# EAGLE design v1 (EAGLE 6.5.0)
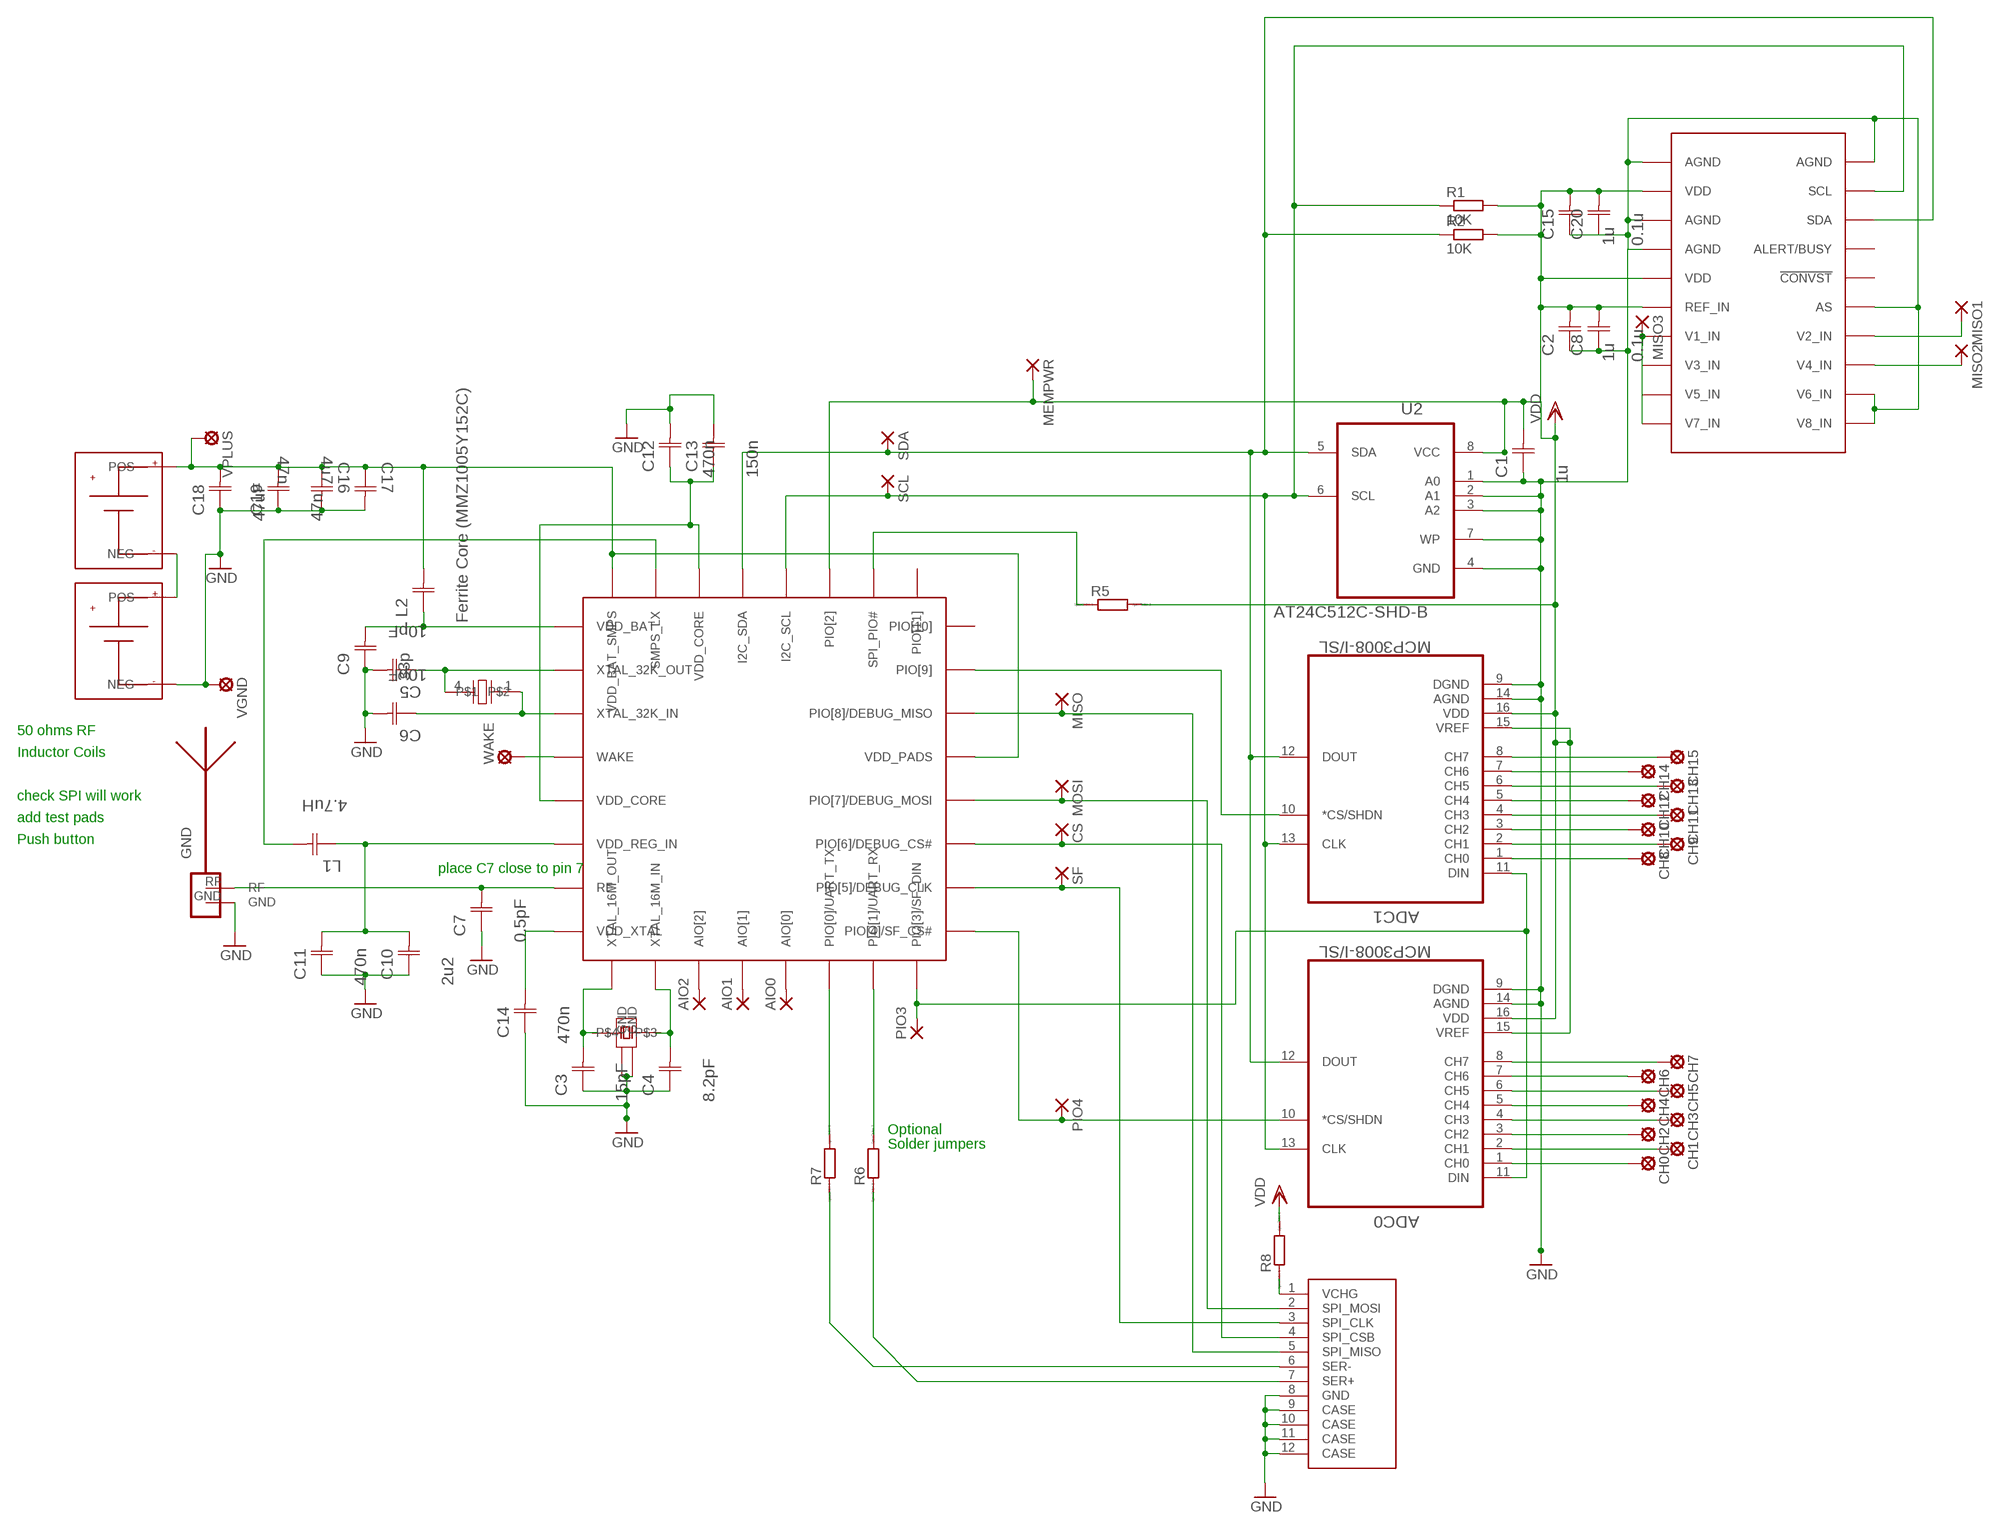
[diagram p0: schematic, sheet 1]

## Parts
ADC0  MCP3008-I/SL  [SOIC127P600X175-16N]
ADC1  MCP3008-I/SL  [SOIC127P600X175-16N]
AIO0  1,6/0,8  [1,6/0,8]
AIO1  1,6/0,8  [1,6/0,8]
AIO2  1,6/0,8  [1,6/0,8]
C1  1u  UQCL2A100JAT2A/500  [CAPC1005X60N]
C2  1u  UQCL2A100JAT2A/500  [CAPC1005X60N]
C3  15pF  UQCL2A150JAT2A/500  [CAPC1005X60N]
C4  8.2pF  UQCL2A8R2CAT2A/500  [CAPC1005X60N]
C5  10pF  UQCL2A100JAT2A/500  [CAPC1005X60N]
C6  10pF  UQCL2A100JAT2A/500  [CAPC1005X60N]
C7  0.5pF  UQCL2A0R5BAT2A/500  [CAPC1005X60N]
C8  0.1u  UQCL2A100JAT2A/500  [CAPC1005X60N]
C9  33p  UQCL2A100JAT2A/500  [CAPC1005X60N]
C10  2u2  UQCL2A100JAT2A/500  [CAPC1005X60N]
C11  470n  UQCL2A100JAT2A/500  [CAPC1005X60N]
C12  470n  UQCL2A100JAT2A/500  [CAPC1005X60N]
C13  150n  UQCL2A100JAT2A/500  [CAPC1005X60N]
C14  470n  UQCL2A100JAT2A/500  [CAPC1005X60N]
C15  1u  UQCL2A100JAT2A/500  [CAPC1005X60N]
C16  47n  UQCL2A1R0BAT2A/500  [CAPC1005X60N]
C17  4u7  UQCL2A1R0BAT2A/500  [CAPC1005X60N]
C18  47uF  0805AA100MAT1A  [CAPC2012X130N]
C19  47n  0805AA100MAT1A  [CAPC2012X130N]
C20  0.1u  UQCL2A100JAT2A/500  [CAPC1005X60N]
CH0  LSP10  [LSP10]
CH1  LSP10  [LSP10]
CH2  LSP10  [LSP10]
CH3  LSP10  [LSP10]
CH4  LSP10  [LSP10]
CH5  LSP10  [LSP10]
CH6  LSP10  [LSP10]
CH7  LSP10  [LSP10]
CH8  LSP10  [LSP10]
CH9  LSP10  [LSP10]
CH10  LSP10  [LSP10]
CH11  LSP10  [LSP10]
CH12  LSP10  [LSP10]
CH13  LSP10  [LSP10]
CH14  LSP10  [LSP10]
CH15  LSP10  [LSP10]
CS  1,6/0,8  [1,6/0,8]
GND  ANTENNA_1LEFT  [SWRA117D_LEFT]
L1  4.7uH  12107C102JAT2A  [CAPC3225X127N]
L2  Ferrite Core (MMZ1005Y152C)  UQCL2A100JAT2A/500  [CAPC1005X60N]
MEMPWR  1,6/0,8  [1,6/0,8]
MISO  1,6/0,8  [1,6/0,8]
MISO1  1,6/0,8  [1,6/0,8]
MISO2  1,6/0,8  [1,6/0,8]
MISO3  1,6/0,8  [1,6/0,8]
MOSI  1,6/0,8  [1,6/0,8]
PIO3  1,6/0,8  [1,6/0,8]
PIO4  1,6/0,8  [1,6/0,8]
R1  10K  R-EU_R0402  [R0402]
R2  10K  R-EU_R0402  [R0402]
R5  RR1206  [R1206]
R6  RR1206  [R1206]
R7  RR1206  [R1206]
R8  RR1206  [R1206]
SCL  1,6/0,8  [1,6/0,8]
SDA  1,6/0,8  [1,6/0,8]
SF  1,6/0,8  [1,6/0,8]
U2  AT24C512C-SHD-B  [SOIC127P798X216-8N]
U$1  CSR1010A05-IQQM-R  [CSR1010A05-IQQM-R]
U$2  8PIN_SMT_CONNECTOR  [8PIN_SMT_CONNECTOR]
U$3  TSX3225  [TSX3225]
U$4  SSP-T7-F  [SSP-T7-F]
U$5  BATTERY_2996  [BATTERY_2996]
U$6  BATTERY_2996  [BATTERY_2996]
U$7  AD7997  [AD7997]
VGND  LSP10  [LSP10]
VPLUS  Vrail  LSP10  [LSP10]
WAKE  Vrail  LSP10  [LSP10]

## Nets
GND: ADC0.9(DGND) ADC0.14(AGND) ADC1.9(DGND) ADC1.14(AGND) C1.2(C1) C2.2(C1) C3.2(C1) C4.2(C1) C5.1(C2) C6.1(C2) C7.2(C1) C8.2(C1) C9.2(C1) C10.2(C1) C11.2(C1) C12.1(C2) C13.1(C2) C14.2(C1) C15.2(C1) C16.1(C2) C17.1(C2) C18.1(C1) C19.1(C1) U2.1(A0) U2.2(A1) U2.3(A2) U2.4(GND) U2.7(WP) U$2.8(GND) U$2.9(CASE) U$2.10(CASE) U$2.11(CASE) U$2.12(CASE) U$3.2(GND) U$3.4(GND) U$5.NEG U$7.P$01(AGND) U$7.P$03(AGND) U$7.P$04(AGND) U$7.P$015(AS) U$7.P$020(AGND) VGND.MP
N$1: ADC0.8(CH7) CH7.MP
N$2: ADC0.7(CH6) CH6.MP
N$3: ADC0.6(CH5) CH5.MP
N$4: ADC0.5(CH4) CH4.MP
N$5: ADC0.4(CH3) CH3.MP
N$6: ADC0.3(CH2) CH2.MP
N$7: ADC0.2(CH1) CH1.MP
N$8: ADC0.1(CH0) CH0.MP
N$9: ADC1.8(CH7) CH15.MP
N$10: ADC1.7(CH6) CH14.MP
N$11: ADC1.6(CH5) CH13.MP
N$12: ADC1.5(CH4) CH12.MP
N$13: ADC1.4(CH3) CH11.MP
N$14: ADC1.3(CH2) CH10.MP
N$15: ADC1.2(CH1) CH9.MP
N$16: ADC1.1(CH0) CH8.MP
N$17: AIO2.1(P) U$1.AIO[2]
N$18: MISO.1(P) U$1.PIO[8]/DEBUG_MISO U$2.5(SPI_MISO)
N$19: L1.2(C2) U$1.SMPS_LX
N$20: R7.1 U$2.6(SER-)
N$23: ADC0.11(DIN) ADC1.11(DIN) PIO3.1(P) U$1.PIO[3]/SF_DIN
N$24: ADC1.10(*CS/SHDN) U$1.PIO[9]
N$25: ADC0.10(*CS/SHDN) PIO4.1(P) U$1.PIO[4]/SF_CS#
N$26: C5.2(C1) U$1.XTAL_32K_OUT U$4.4
N$27: C6.2(C1) U$1.XTAL_32K_IN U$4.1
N$29: C3.1(C2) U$1.XTAL_16M_OUT
N$30: C4.1(C2) U$1.XTAL_16M_IN
N$31: CS.1(P) U$1.PIO[6]/DEBUG_CS# U$2.4(SPI_CSB)
N$32: C9.1(C2) L2.2(C1) U$1.VDD_BAT
N$33: AIO1.1(P) U$1.AIO[1]
N$34: C16.2(C1) C17.2(C1) C18.2(C2) C19.2(C2) L2.1(C2) U$1.VDD_BAT_SMPS U$1.VDD_PADS U$6.POS@1(POS) VPLUS.MP
N$35: C14.1(C2) U$1.VDD_XTAL
N$36: R6.1 U$2.7(SER+)
N$37: R7.2 U$1.PIO[0]/UART_TX
N$38: R6.2 U$1.PIO[1]/UART_RX
N$39: C10.1(C2) C11.1(C2) L1.1(C1) U$1.VDD_REG_IN
N$40: R8.1 U$2.1(VCHG)
N$41: AIO0.1(P) U$1.AIO[0]
N$43: C7.1(C2) U$1.RF
N$45: R5.1 U$1.SPI_PIO#
N$48: U$5.POS@1(POS) U$6.NEG
N$49: U$1.WAKE WAKE.MP
N$50: MOSI.1(P) U$1.PIO[7]/DEBUG_MOSI U$2.2(SPI_MOSI)
N$51: SF.1(P) U$1.PIO[5]/DEBUG_CLK U$2.3(SPI_CLK)
N$86: MISO1.1(P) U$7.P$014(V2_IN)
N$87: MISO2.1(P) U$7.P$013(V4_IN)
N$88: MISO3.1(P) U$7.P$07(V1_IN) U$7.P$010(V7_IN)
N$90: U$7.P$011(V8_IN) U$7.P$012(V6_IN)
SCL: ADC0.13(CLK) ADC1.13(CLK) R1.1 SCL.1(P) U2.6(SCL) U$1.I2C_SCL U$7.P$019(SCL)
SDA: ADC0.12(DOUT) ADC1.12(DOUT) R2.1 SDA.1(P) U2.5(SDA) U$1.I2C_SDA U$7.P$018(SDA)
VDD: ADC0.15(VREF) ADC0.16(VDD) ADC1.15(VREF) ADC1.16(VDD) C1.1(C2) C2.1(C2) C8.1(C2) C15.1(C2) C20.1(C2) MEMPWR.1(P) R1.2 R2.2 R5.2 R8.2 U2.8(VCC) U$1.PIO[2] U$7.P$02(VDD) U$7.P$05(VDD) U$7.P$06(REF_IN)
VDD_CORE: C12.2(C1) C13.2(C1) U$1.VDD_CORE U$1.VDD_CORE@1(VDD_CORE)
Unconnected: C20.2(C1) GND.GND GND.RF U$1.PIO[10] U$1.PIO[11] U$3.1 U$3.3 U$7.P$08(V3_IN) U$7.P$09(V5_IN) U$7.P$016(!CONVST) U$7.P$017(ALERT/BUSY)

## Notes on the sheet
- 50 ohms RF
- Inductor Coils
- check SPI will work
- add test pads
- Push button
- place C7 close to pin 7
- Optional
- Solder jumpers

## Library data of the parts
ADC0 ADC1 = Microchip_By_element14_Batch_1:MCP3008-I/SL: 10BIT ADC, 8 CH, SPI, SMD; MPN: MCP3008-I/SL; OC_FARNELL: 1292241; OC_NEWARK: 19C7201; PACKAGE: SOIC16; SUPPLIER: Microchip
AIO0 AIO1 AIO2 CS MEMPWR MISO MISO1-MISO3 MOSI PIO3 PIO4 SCL SDA SF = wirepad:1,6/0,8: THROUGH-HOLE PAD
C1 C2 C8-C15 C20 L2 = AVX_By_element14_Batch_1:UQCL2A100JAT2A/500: Capacitor 0402; MPN: UQCL2A100JAT2A/500; OC_FARNELL: -; OC_NEWARK: 32T8791; SUPPLIER: AVX; TOLERANCE: ±5%; VALUE: 10pF; VOLTAGERATING: 200V
C3 = AVX_By_element14_Batch_1:UQCL2A150JAT2A/500: Capacitor 0402; MPN: UQCL2A150JAT2A/500; OC_FARNELL: -; OC_NEWARK: 32T8795; SUPPLIER: AVX; TOLERANCE: ±5%; VOLTAGERATING: 200V
C4 = AVX_By_element14_Batch_1:UQCL2A8R2CAT2A/500: Capacitor 0402; MPN: UQCL2A8R2CAT2A/500; OC_FARNELL: -; OC_NEWARK: 32T8828; SUPPLIER: AVX; TOLERANCE: ±.25 pF; VOLTAGERATING: 200V
C5 C6 = AVX_By_element14_Batch_1:UQCL2A100JAT2A/500: Capacitor 0402; MPN: UQCL2A100JAT2A/500; OC_FARNELL: -; OC_NEWARK: 32T8791; SUPPLIER: AVX; TOLERANCE: ±5%; VOLTAGERATING: 200V
C7 = AVX_By_element14_Batch_1:UQCL2A0R5BAT2A/500: Capacitor 0402; MPN: UQCL2A0R5BAT2A/500; OC_FARNELL: -; OC_NEWARK: 32T8767; SUPPLIER: AVX; TOLERANCE: ±.1 pF; VOLTAGERATING: 200V
C16 C17 = AVX_By_element14_Batch_1:UQCL2A1R0BAT2A/500: Capacitor 0402; MPN: UQCL2A1R0BAT2A/500; OC_FARNELL: -; OC_NEWARK: 32T8778; SUPPLIER: AVX; TOLERANCE: ±.1 pF; VALUE: 1pF; VOLTAGERATING: 200V
C18 C19 = AVX_By_element14_Batch_1:0805AA100MAT1A: Capacitor 0805; MPN: 0805AA100MAT1A; OC_FARNELL: -; OC_NEWARK: 18M6883; SUPPLIER: AVX; TOLERANCE: ±20%; VALUE: 10pF; VOLTAGERATING: 1000V (1kV)
CH0 CH1-CH15 VGND VPLUS WAKE = solpad:LSP10: SOLDER PAD
GND = ant-planar-1:ANTENNA_1
L1 = AVX_By_element14_Batch_1:12107C102JAT2A: Capacitor 1210; MPN: 12107C102JAT2A; OC_FARNELL: -; OC_NEWARK: 56J0850; SUPPLIER: AVX; TOLERANCE: ±5%; VALUE: 1000PF; VOLTAGERATING: 500V
R1 R2 = rcl:R-EU_: RESISTOR, European symbol
R5-R8 = eagle-ltspice:R: RESISTOR, European symbol; SPICEMODEL: NONE; SPICEPREFIX: R
U2 = ATMEL-AT24C512C-SHD-B:AT24C512C-SHD-B: EEPROM, SERIAL, 512K (64KX8), 8SOIC-Wide; MPN: AT24C512C-SHD-B; OC_FARNELL: 1972003; OC_NEWARK: 68T4124; PACKAGE: 8SOIC-Wide; SUPPLIER: ATMEL
U$1 = CSR1010A05:CSR1010A05-IQQM-R
U$2 = MINI_SMT_8_PIN_CONNECTOR:8PIN_SMT_CONNECTOR
U$3 = TSX3225:TSX3225
U$4 = SSP-T7-F:SSP-T7-F
U$5 U$6 = BATTERY_2996:BATTERY_2996
U$7 = AD7997:AD7997

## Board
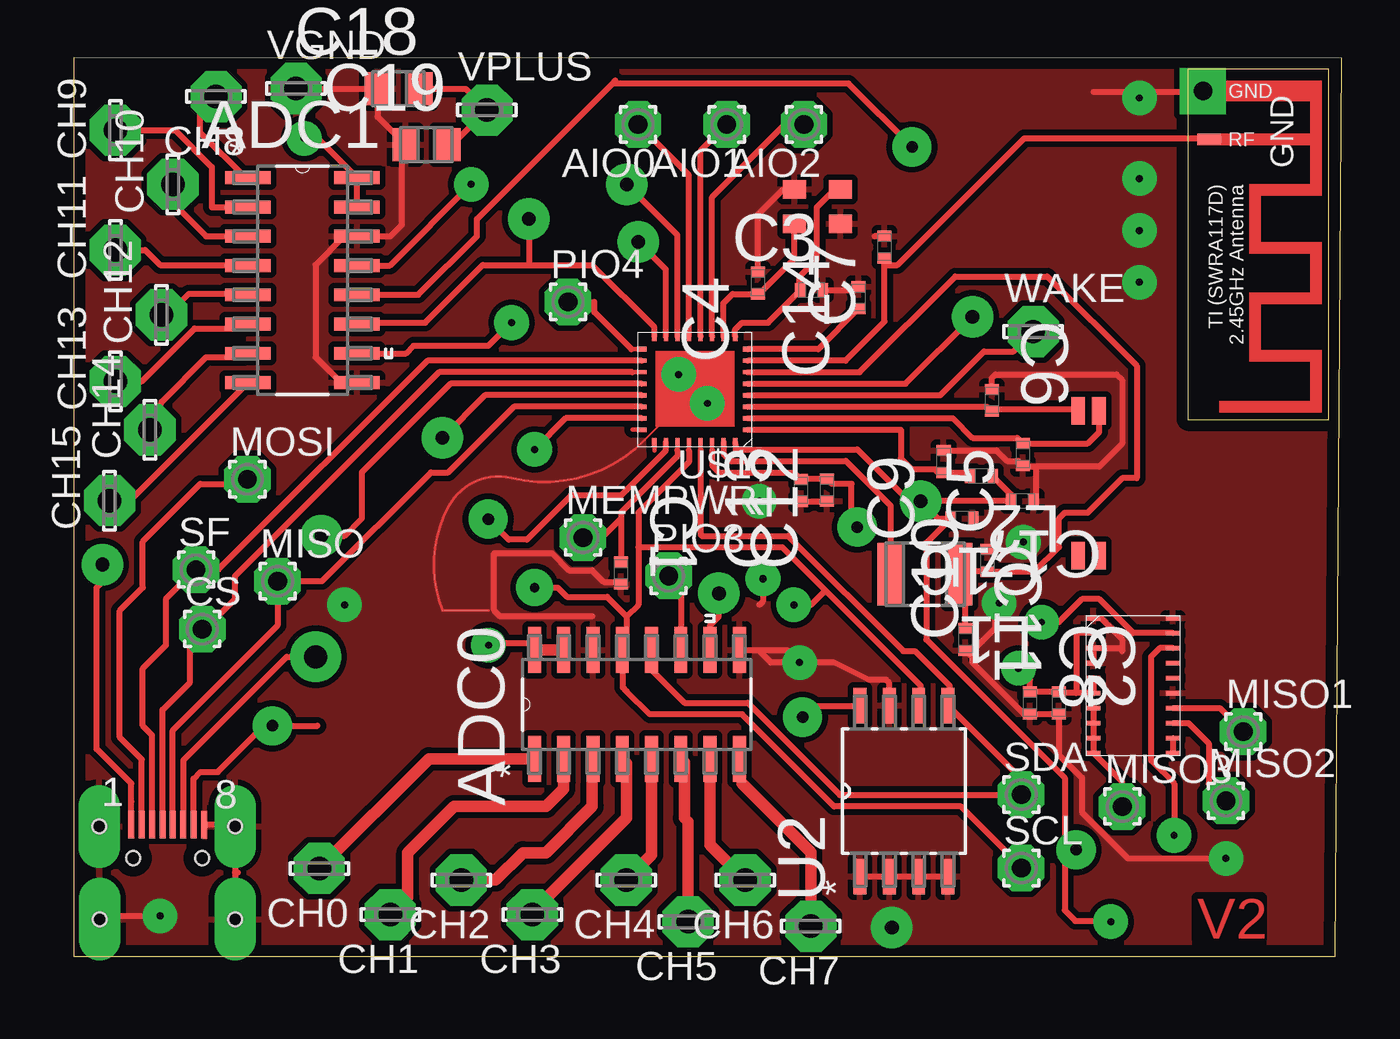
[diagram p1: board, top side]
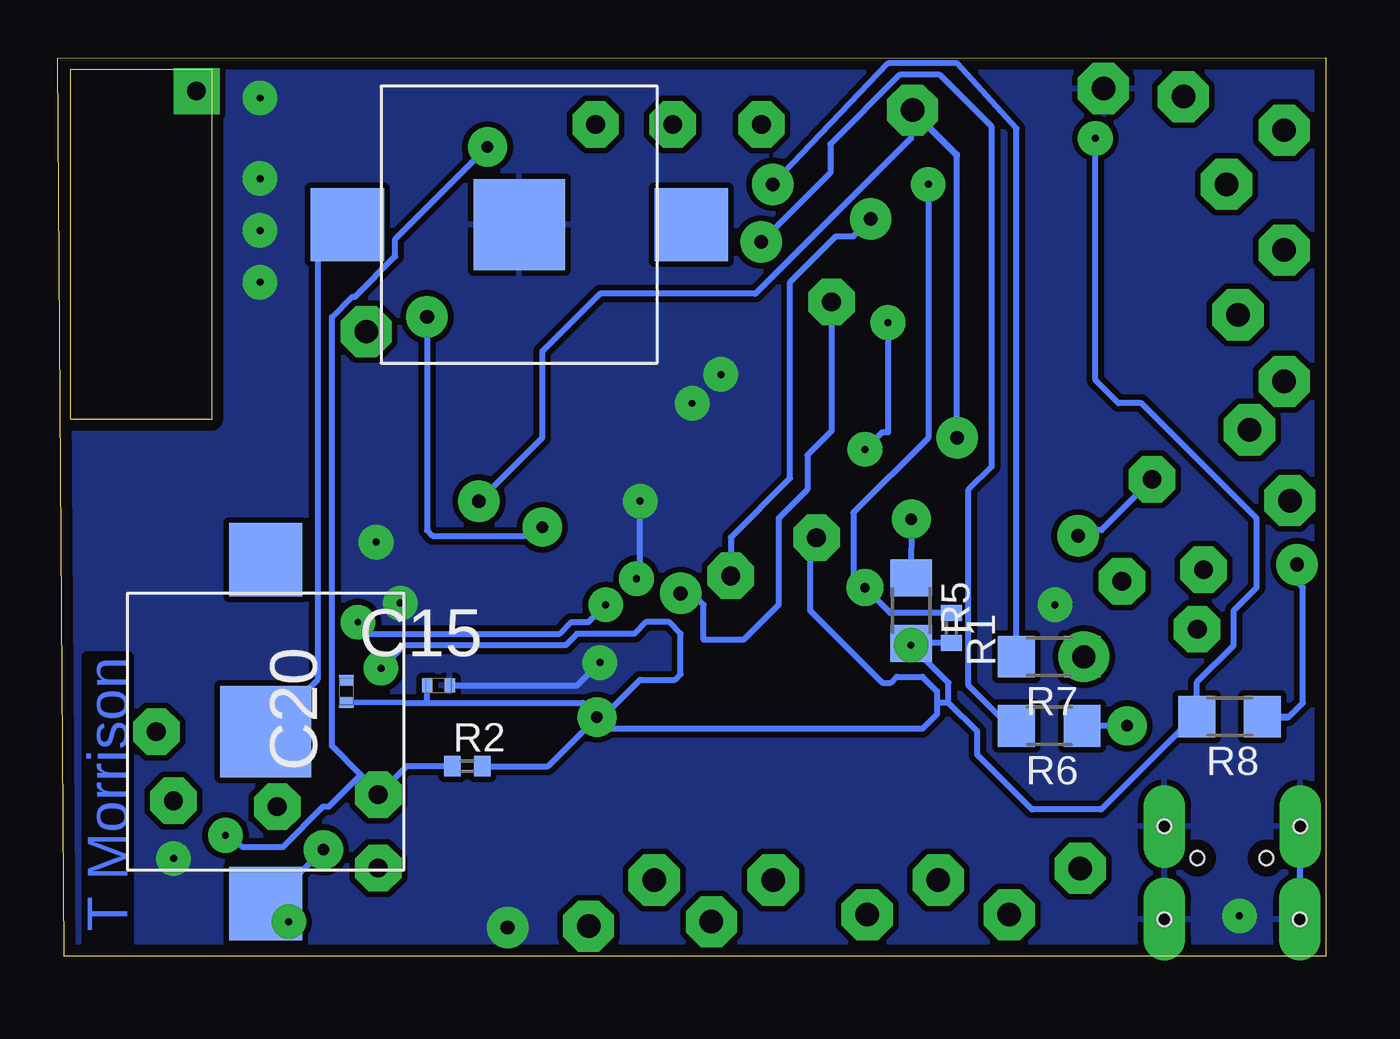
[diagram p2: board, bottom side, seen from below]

Size 55.04 x 38.99 mm. Coordinates in mm from the lower left corner, seen from the top.
Outline: 0.01,0 54.76,0 55.04,38.98 0,38.99 0.01,0
Copper layers (1*16): Top 0.035mm / dielectric 1.5mm / Bottom 0.035mm
Design rules "DRC *": minimum track width 0.25mm, minimum drill 0.5mm, track to track 0.25mm, track to pad 0.25mm, pad to pad 0.15mm, via to via 0.25mm, smd to smd 0.15mm, copper to edge 0.5mm, drill to drill 0.4mm, minimum pad ring 0.6mm, minimum via ring 0.6mm, stop-mask expansion 4mil, vias tented up to drill 0mil, thermal gap 10mil

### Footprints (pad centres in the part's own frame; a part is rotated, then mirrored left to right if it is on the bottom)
SOIC127P600X175-16N = smd 1.981 x 0.559: 1 -2.362,4.445; 2 -2.362,3.175; 3 -2.362,1.905; 4 -2.362,0.635; 5 -2.362,-0.635; 6 -2.362,-1.905; 7 -2.362,-3.175; 8 -2.362,-4.445; 9 2.362,-4.445; 10 2.362,-3.175; 11 2.362,-1.905; 12 2.362,-0.635; 13 2.362,0.635; 14 2.362,1.905; 15 2.362,3.175; 16 2.362,4.445
1,6/0,8 = drill 0.813 pad 1.6 octagon: 1 0,0
CAPC1005X60N = smd 0.457 x 0.61: 1 -0.483,0; 2 0.483,0
CAPC2012X130N = smd 1.118 x 1.448: 1 -0.914,0; 2 0.914,0
LSP10 = drill 1.016 pad 2.159 octagon: MP 0,0
SWRA117D_LEFT = drill 0.8 square: GND 0.45,0.25 | smd 0.508 x 1.016: RF 2.55,0.51
CAPC3225X127N = smd 1.118 x 2.692: 1 -1.499,0; 2 1.499,0
R0402 = smd 0.7 x 0.9: 1 -0.65,0; 2 0.65,0
R1206 = smd 1.6 x 1.803: 1 -1.422,0; 2 1.422,0
SOIC127P798X216-8N = smd 1.549 x 0.559: 1 -3.708,1.905; 2 -3.708,0.635; 3 -3.708,-0.635; 4 -3.708,-1.905; 5 3.708,-1.905; 6 3.708,-0.635; 7 3.708,0.635; 8 3.708,1.905
CSR1010A05-IQQM-R = smd 0.186 x 0.4: AIO[0] -0.2,-0.9; AIO[1] -0.7,-0.9; AIO[2] -1.2,-0.9; I2C_SCL -0.2,3.7; I2C_SDA -0.7,3.7; PIO[0]/UART_TX 0.3,-0.9; PIO[1]/UART_RX 0.8,-0.9; PIO[2] 0.3,3.7; SMPS_LX -1.7,3.7; SPI_PIO# 0.8,3.7; VDD_CORE@1 -1.2,3.7; XTAL_16M_IN -1.7,-0.9 | smd 0.2 x 0.4: PIO[3]/SF_DIN 1.3,-0.9; PIO[11] 1.3,3.7; VDD_BAT_SMPS -2.2,3.7; XTAL_16M_OUT -2.2,-0.9 | smd 0.4 x 0.2: PIO[4]/SF_CS# 1.85,-0.35; PIO[10] 1.85,3.15; VDD_BAT -2.75,3.15; VDD_XTAL -2.75,-0.35 | smd 0.4 x 0.186: PIO[5]/DEBUG_CLK 1.85,0.15; PIO[6]/DEBUG_CS# 1.85,0.65; PIO[7]/DEBUG_MOSI 1.85,1.15; PIO[8]/DEBUG_MISO 1.85,2.15; PIO[9] 1.85,2.65; RF -2.75,0.15; VDD_CORE -2.75,1.15; VDD_PADS 1.85,1.65; VDD_REG_IN -2.75,0.65; WAKE -2.75,1.65; XTAL_32K_IN -2.75,2.15; XTAL_32K_OUT -2.75,2.65
8PIN_SMT_CONNECTOR = smd 0.26 x 1.2: 1 -1.32,2.83; 2 -0.87,2.83; 3 -0.42,2.83; 4 0.03,2.83; 5 0.48,2.83; 6 0.93,2.83; 7 1.38,2.83; 8 1.83,2.83 | drill 0.6 long: 9 3.18,2.755; 10 3.18,-1.27; 11 -2.695,-1.27; 12 -2.72,2.755 | hole 0.6: -2.72,2.755; -2.695,-1.27; 3.18,-1.27; 3.18,2.755; 1.755,1.38; -1.245,1.38
TSX3225 = smd 1 x 0.8: 1 -1,-0.75; 2 1,-0.75; 3 1,0.75; 4 -1,0.75
SSP-T7-F = smd 1.2 x 0.6: 1 -0.6,0.3; 2 5.7,0.3; 3 5.7,1.2; 4 -0.6,1.2
BATTERY_2996 = smd 3.96 x 3.96: NEG 0,0 | smd 3.18 x 3.18: POS@1 -7.463,0; POS@2 7.463,0
AD7997 = smd 0.6 x 0.2: P$01 -1.75,2.925; P$02 -1.75,2.275; P$03 -1.75,1.625; P$04 -1.75,0.975; P$05 -1.75,0.325; P$06 -1.75,-0.325; P$07 -1.75,-0.975; P$08 -1.75,-1.625; P$09 -1.75,-2.275; P$010 -1.75,-2.925; P$011 1.7,-2.925; P$012 1.7,-2.275; P$013 1.7,-1.625; P$014 1.7,-0.975; P$015 1.7,-0.325; P$016 1.7,0.325; P$017 1.7,0.975; P$018 1.7,1.625; P$019 1.7,2.275; P$020 1.7,2.925

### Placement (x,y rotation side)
ADC0  24.45,10.93 90 top
ADC1  9.94,29.34 0 top
AIO0  24.5,36.1 180 top
AIO1  28.35,36.1 180 top
AIO2  31.7,36.1 180 top
C1  23.76,16.63 270 top
C2  42.76,11 270 top
C3  32.03,28.9 0 top
C4  29.71,29.22 90 top
C5  41.19,21.77 90 top
C6  39.85,24.13 270 top
C7  35.19,30.78 90 top
C8  41.51,11 270 top
C9  37.76,21.47 90 top
C10  39.66,17.18 90 top
C11  38.7,13.75 270 top
C12  32.69,20.23 90 top
C13  31.57,20.22 90 top
C14  34.07,28.58 90 top
C15  38.51,11.75 0 bottom
C16  38.55,19 180 top
C17  41.17,19.75 180 top
C18  14.1,37.65 0 top
C19  15.32,35.22 0 top
C20  42.51,11.5 90 bottom
CH0  10.67,3.81 180 top
CH1  13.75,1.81 180 top
CH2  16.83,3.31 180 top
CH3  19.91,1.81 180 top
CH4  23.99,3.31 180 top
CH5  26.67,1.5 180 top
CH6  29.15,3.31 180 top
CH7  32,1.31 180 top
CH8  6.19,37.31 180 top
CH9  1.82,35.85 90 top
CH10  4.32,33.5 90 top
CH11  1.82,30.65 90 top
CH12  3.82,27.84 90 top
CH13  1.82,24.95 90 top
CH14  3.32,22.85 90 top
CH15  1.57,19.77 90 top
CS  5.59,14.2 0 top
GND  48.76,38 270 top
L1  36.95,16.58 180 top
L2  39.4,20.85 180 top
MEMPWR  22.11,18.17 0 top
MISO  8.86,16.28 0 top
MISO1  50.76,9.75 0 top
MISO2  50.01,6.75 0 top
MISO3  45.51,6.5 0 top
MOSI  7.55,20.7 0 top
PIO3  25.82,16.51 0 top
PIO4  21.46,28.4 0 top
R1  16.26,14.25 270 bottom
R2  37.26,8.25 0 bottom
R5  18.01,15 270 bottom
R6  12.01,10 180 bottom
R7  12.01,13 180 bottom
R8  4.18,10.4 180 bottom
SCL  41.13,3.83 0 top
SDA  41.13,7.02 0 top
SF  5.32,16.78 0 top
U2  36.04,7.17 90 top
U$1  26.51,26 180 top
U$2  3.83,2.88 0 top
U$3  32.28,32.54 0 top
U$4  43.29,23.08 270 top
U$5  35.01,31.75 0 bottom
U$6  46.01,9.75 90 bottom
U$7  46.01,11.75 0 top
VGND  9.66,37.66 0 top
VPLUS  17.94,36.73 0 top
WAKE  41.65,27.11 0 top

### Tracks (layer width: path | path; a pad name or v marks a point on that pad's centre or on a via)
GND  (via drill 0.3, 0.6)
  Top 0.1: 24.77,22.4 25.58,23.2 | 25.58,23.2 | 25.58,23.2 24.78,22.39 arc-59 19.01,20.75 arc76 16.26,19.5 arc49 16.01,15 18.01,15
  Top 0.25: U2.1 U2.2 U2.4 | C4.2 29.69,29.71 29.69,32.19 30.76,33.25 31.24,33.25 U$3.4 | VGND.MP 12.95,37.66 C18.1 13.19,36.44 C19.1 14.26,35.08 14.26,31.75 13.75,31.25 ADC1.14 11.75,31.25 10.51,30 10.51,26 11.51,25 11.63,25 | 11.63,25 12.19,25 ADC1.9 11.63,25 | 1.26,1.5 1.16,1.5 | C9.2 40.05,21.95 40.51,21.5 40.98,21.5 C5.1 41.23,21.25 41.76,21.25 | 11.63,25 11.63,24.91 | C17.1 41.63,19.62 41.65,19.62 | C17.1 41.63,19.75 C17.1 | 41.76,21.25 44.51,21.25 45.51,22.25 45.51,25 45.26,25.25 40.01,25.25 39.85,25.09 C6.1 | 41.76,21.25 41.76,19.86 C17.1 | C12.1 32.68,19.74 C13.1 31.55,19.75 v29.76,19.75 | 22.51,14.75 18.51,14.75 18.26,15 18.26,17.5 20.76,17.5 21.51,16.75 22.51,16.75 23.01,16.25 23.65,16.25 C1.2 | C3.2 33.91,28.91 C14.2 | 6.94,5.71 U$2.8 | U$2.9 7.01,3.62 | 7.01,3.62 U$2.10 | 49.01,37.5 44.26,37.5 | C7.2 35.18,31.25 34.76,31.25 | 7.13,3.62 7.01,3.62 | v50.01,4.25 45.76,4.25 43.76,6.25 43.76,7.75 42.76,8.75 C2.2 C8.2 41.24,10.52 39.01,12.75 39.01,12.96 C11.2 39.02,13.27 40.01,14.25 40.01,15.16 v40.17,15.33 | U2.7 35.4,11.86 35.26,12 34.51,12 33.01,12.75 v31.51,12.75 | 25.58,23.2 26.71,23.2 v27.51,24 27.26,24 26.26,25 v26.26,25.25 | U$7.P$01 44.58,14.68 45.51,13.75 45.51,13.25 45.38,13.38 U$7.P$03 U$7.P$04 | ADC0.9 30.96,13.29 v31.51,12.75 | v29.92,16.38 29.92,15.41 29.76,15.25 | v31.51,12.75 30.26,12.75 29.76,13.25 | 1.16,1.5 1.41,1.75 v3.76,1.75 | 1.16,1.5 1.14,1.52 U$2.11
  Top 0.5: 6.94,5.71 U$2.9
  Bottom 0.25: v29.76,19.75 29.76,16.54 v29.92,16.38 | C15.2 32.51,11.75 v31.51,12.75 | U$2.11 1.11,1.64 U$2.12
  other vias: 46.26,37.25 46.26,33.75 46.26,31.5 46.26,29.25 11.76,15.25 35.51,1.25 41.22,17.98
  pour Top: 0.01,39 55.01,39 54.76,0 0.01,0
  pour Bottom: 0.01,0 54.76,0 55.01,39 0.01,39
N$1
  Top 0.25: 29.01,7.5 29.01,8.5 ADC0.8
  Top 0.5: CH7.MP 32,4.51 29.01,7.5
N$2
  Top 0.5: ADC0.7 27.62,4.83 CH6.MP
N$3
  Top 0.5: ADC0.6 26.51,8.41 26.51,6 26.67,5.84 CH5.MP
N$4
  Top 0.5: ADC0.5 25.08,4.41 CH4.MP
N$5
  Top 0.5: CH3.MP 19.91,1.9 24.01,6 24.01,8.37 ADC0.4
N$6
  Top 0.25: 22.51,7.5 22.51,8.5 ADC0.3
  Top 0.5: CH2.MP 18.32,3.31 19.51,4.5 20.51,4.5 22.51,6.5 22.51,7.5
N$7
  Top 0.5: ADC0.2 21.27,7.26 20.51,6.5 16.51,6.5 14.51,4.5 14.51,2.57 CH1.MP
N$8
  Top 0.5: CH0.MP 15.42,8.57 ADC0.1
N$9
  Top 0.25: CH15.MP 2.45,19.77 ADC1.8
N$10
  Top 0.25: CH14.MP 3.82,24.06 5.76,26 7.41,26 ADC1.7
N$11
  Top 0.25: CH13.MP 2.96,24.95 5.26,27.25 7.39,27.25 ADC1.6
N$12
  Top 0.25: CH12.MP 4.09,27.84 5.01,28.75 7.53,28.75 ADC1.5
N$13
  Top 0.25: CH11.MP 3.11,30.65 3.76,30 7.55,30 ADC1.4
N$14
  Top 0.25: CH10.MP 4.32,32.69 5.76,31.25 ADC1.3
N$15
  Top 0.25: CH9.MP 4.41,35.85 6.01,34.25 6.01,32.5 7.56,32.5 ADC1.2
N$16
  Top 0.25: ADC1.1 7.47,33.78 5.51,35.75 5.51,36.63 CH8.MP
N$17
  Top 0.25: U$1.AIO[2] 27.71,32.95 30.76,36 31.6,36 AIO2.1
N$18
  Top 0.25: U$2.5 4.31,9.8 8.86,14.35 MISO.1 10.79,16.28 15.51,21 16.26,21 19.11,23.85 U$1.PIO[8]/DEBUG_MISO
N$19
  Top 0.25: L1.2 35.45,19.56 33.51,21.5 28.51,21.5 28.21,21.8 U$1.SMPS_LX
N$20  (via drill 1)
  Top 0.25: U$2.6 4.78,6.73 4.78,8.52 9.26,13 v10.51,13 R7.1
  Bottom 0.25: v10.51,13 R7.1
N$21  (via drill 0.3)
  other vias: 31.26,15.25
N$23  (via drill 0.6)
  Top 0.25: 26.32,13.32 ADC0.11 26.35,15.98 PIO3.1 | ADC1.11 12.36,27.5 15.26,27.5 17.76,30 19.76,30 | 19.76,30 22.51,30 25.21,27.3 U$1.PIO[3]/SF_DIN | v19.76,32 19.76,30
  Bottom 0.25: v19.76,32 20.51,31.25 21.26,31.25 23.26,29.25 23.26,20.75 25.82,18.18 PIO3.1
N$24  (via drill 0.3)
  Top 0.25: ADC1.10 14.42,26.16 14.76,26.5 18.01,26.5 v19.01,27.5 | v20.01,22 21.36,23.35 U$1.PIO[9]
  Bottom 0.25: v19.01,27.5 19.01,22.75 19.26,22.75 v20.01,22
N$25  (via drill 0.6)
  Top 0.25: PIO4.1 22.61,28.4 22.61,27.95 24.21,26.35 | ADC0.10 27.62,14.37 28.01,14.75 v28.01,15.75
  Bottom 0.25: PIO4.1 21.46,22.8 22.51,21.75 22.51,20.25 23.76,19 23.76,15.25 25.26,13.75 27.01,13.75 27.01,15.25 27.51,15.75 v28.01,15.75
N$26
  Top 0.25: U$4.4 44.51,23.66 44.51,22.75 44.01,22.26 C5.2 40.95,22.5 39.01,22.5 38.16,23.35 U$1.XTAL_32K_OUT
N$27
  Top 0.25: U$4.1 43.51,23.75 39.88,23.75 C6.2 39.65,23.85 U$1.XTAL_32K_IN
N$28  (via drill 0.3)
  other vias: 41.01,12.5
N$29
  Top 0.25: U$1.XTAL_16M_OUT 28.71,27.2 29.01,27.5 30.14,27.5 C3.1
N$30
  Top 0.25: C4.1 28.6,28.74 28.2,28.34 28.2,27 U$1.XTAL_16M_IN
N$31
  Top 0.25: U$2.4 3.86,10.7 5.05,11.89 5.05,13.67 CS.1 5.71,14.2 7.01,15.5 7.01,16.5 15.86,25.35 24.26,25.35
N$32
  Top 0.25: L2.2 38.78,20.99 C9.1 37.74,21 37.51,21 37.38,21.12 36.38,21.12 35.89,21.61 35.89,22.85 U$1.VDD_BAT
N$33
  Top 0.25: U$1.AIO[1] 27.21,34.96 AIO1.1
N$34  (via drill 0.5, 0.6)
  Top 0.25: C18.2 17.02,37.65 VPLUS.MP 16.43,35.22 C19.2 | v16.01,22.5 17.86,24.35 U$1.VDD_PADS | v36.76,19.75 36.26,19.75 34.01,22 28.76,22 U$1.VDD_BAT_SMPS | v36.76,19.75 37.51,19 C16.2 37.01,17.94 37.01,13.75 43.01,7.75 43.01,4.62 | 36.78,19.75 v36.76,19.75 | 43.01,4.62 43.01,2 43.47,1.54 45.01,1.54 | v36.76,19.75 C17.2 40.68,20.04 L2.1 | 43.01,4.62 v43.51,4.62
  Bottom 0.25: 16.01,34.75 16.01,34.79 VPLUS.MP | v16.01,22.5 16.01,34.75 | 16.01,34.75 18.01,36.75 18.01,35.5 24.76,28.75 31.51,28.75 34.01,26.25 34.01,22.5 v36.76,19.75 | 45.01,1.54 45.76,2.29 U$6.POS@1 45.76,2.38 v43.51,4.62
N$35
  Top 0.25: C14.1 32.32,26.35 U$1.VDD_XTAL
N$36  (via drill 0.5)
  Top 0.25: U$2.7 5.21,7.71 5.51,8 6.26,8 8.26,10 v8.63,10 R6.1
  Bottom 0.25: v8.63,10 R6.1
N$37  (via drill 0.6)
  Top 0.25: v24.01,33.5 26.21,31.3 U$1.PIO[0]/UART_TX
  Bottom 0.25: R7.2 13.43,35.92 16.01,38.75 19.01,38.75 v24.01,33.5
N$38  (via drill 0.6)
  Top 0.25: v24.51,31 25.71,29.8 U$1.PIO[1]/UART_RX
  Bottom 0.25: R6.2 13.76,10 15.51,11.75 15.51,20.25 14.51,21.25 14.51,36 16.76,38.25 18.51,38.25 21.51,35.25 21.51,34 v24.51,31
N$39
  Top 0.25: C11.1 38.7,15.75 | 38.7,15.75 38.7,16.33 L1.1 | 38.72,15.73 38.7,15.75 | L1.1 38.45,16.06 38.76,15.75 | U$1.VDD_REG_IN 34.11,25.35 38.26,29.5 42.26,29.5 46.13,25.62 46.13,20.75 45.51,20.75 44.01,19.25 43.01,19.25 42.76,19 42.76,17.75 41.7,16.69 C10.1 38.56,16.69 L1.1
N$40  (via drill 0.6)
  Top 0.25: U$2.1 2.51,6.72 2.51,7.5 1.01,9 1.01,16 1.26,16.25 v1.26,17
  Bottom 0.25: 1.6,10.4 R8.1 2.73,10.38 1.63,10.38 1.6,10.4 | 1.6,10.4 1.01,11 1.01,16 1.26,16.25 v1.26,17
N$41
  Top 0.25: U$1.AIO[0] 26.71,33.89 AIO0.1
N$43
  Top 0.25: C7.1 35.19,27.55 33.5,25.85 U$1.RF
N$45  (via drill 0.5)
  Top 0.25: v17.99,18.98 18.88,18.09 19.67,18.09 21.58,20 23.76,20 25.71,21.95 U$1.SPI_PIO#
  Bottom 0.25: v17.99,18.98 18.01,16.5 R5.1
N$46  (via drill 0.3)
  other vias: 29.91,16.39
N$48
  Bottom 0.25: U$5.POS@1 43.76,32.25 43.76,12 U$6.NEG
N$49
  Top 0.25: WAKE.MP 40.79,26.25 39.51,26.25 37.61,24.35 U$1.WAKE
N$50  (via drill 0.6)
  Top 0.25: 2.96,6.71 U$2.2 2.96,8.54 2.01,9.5 2.01,15 3.01,16 3.01,18 5.51,20.5 7.35,20.5 MOSI.1 | v10.76,18.25 11.76,18.25 12.51,19 12.51,21 16.36,24.85 U$1.PIO[7]/DEBUG_MOSI
  Bottom 0.25: MOSI.1 9.75,18.5 10.01,18.5 10.26,18.25 v10.76,18.25
N$51
  Top 0.25: U$2.3 3.41,9.6 3.01,10 3.01,12.5 4.01,13.5 4.01,15.5 5.29,16.78 SF.1 6.29,16.78 15.36,25.85 U$1.PIO[5]/DEBUG_CLK
N$73  (via drill 0.6)
  other vias: 10.76,18.25
N$79
  Top 0.25: 31.26,32 31.26,30.25 29.76,28.75
N$84
  Top 0.25: 35.26,30 35.76,30 41.26,35.5 49.01,35.5
N$85
  Top 0.25: 31.51,29 31.51,29.5 32.26,30.25 32.26,32.5 33.01,33.25 33.26,33.25
N$86
  Top 0.25: U$7.P$014 49.73,10.78 MISO1.1
N$87
  Top 0.25: U$7.P$013 48.38,10.12 49.26,9.25 49.26,7.5 MISO2.1
N$88
  Top 0.25: MISO3.1 45.51,7.58 U$7.P$010 U$7.P$07
N$89  (via drill 0.3)
  other vias: 45.01,1.5
N$90
  Top 0.25: U$7.P$012 U$7.P$011
SCL  (via drill 0.3, 0.4)
  Top 0.25: SCL.1 41.13,3.88 38.51,6.5 33.01,6.5 29.01,10.5 25.01,10.5 24.01,11.5 24,11.5 23.84,11.66 23.84,13.26 ADC0.13 24.01,13.49 24.01,14.75 | 24.51,17.75 24.51,19.25 26.71,21.45 26.71,21.95 | 24.51,17.75 24.51,15.25 24.01,14.75 | 36.67,11.34 U2.6 36.76,10.96 36.76,11.75 32.63,15.88 | 24.51,17.75 30.76,17.75 32.63,15.88 | ADC1.13 13.73,29.98 v17.26,33.5 | 24.01,14.75 23.16,15.6 21.41,15.6 21.01,16 v20.01,16 | U$7.P$019 45.98,14.03 44.51,15.5 43.76,15.5 42.76,14.5 v42.01,14.5 | v31.26,15.25 32.01,15.25 32.63,15.88
  Bottom 0.25: v17.26,33.5 17.26,22.5 20.51,19.25 20.51,16.5 v20.01,16 18.91,14.9 R1.1 | v42.01,14.5 41.51,14 33.26,14 32.76,14.5 32.01,14.5 v31.26,15.25
SDA  (via drill 0.3, 0.5)
  Top 0.25: ADC0.12 25.08,12.43 26.51,11 29.26,11 33.26,7 41.11,7 SDA.1 41.13,7.69 U2.5 38.01,10.94 38.01,11.75 36.51,13.25 36.01,13.25 31.01,18.25 27.26,18.25 27.21,18.3 27.21,21.95 | ADC1.12 14.96,28.7 17.51,31.25 17.51,32 23.44,37.94 | 23.44,37.94 23.51,38 | v36.38,35.12 33.63,37.88 23.51,37.88 23.44,37.94 | U$7.P$018 47.13,13.38 46.76,13 46.76,8.5 47.76,7.5 v47.76,5.25
  Bottom 0.25: v36.38,35.12 40.38,31.12 40.38,30.38 42.13,28.62 42.26,28.62 43.13,27.75 43.13,9.12 41.88,7.88 | 41.88,7.88 41.13,7.12 SDA.1 39.9,8.25 R2.1 | v47.76,5.25 47.01,4.75 45.26,4.75 43.51,6.5 43.26,6.5 41.88,7.88
VDD  (via drill 0.3, 0.5)
  Top 0.25: ADC1.15 ADC1.16 10.58,35.5 v10.01,35.5 | ADC0.16 19.72,13.58 R5.2 v18.01,13.5 | 23.76,19 23.76,19.25 26.21,21.7 26.21,21.95 | 23.76,19 C1.1 | 23.76,19 22.93,18.17 MEMPWR.1 | v31.63,10.38 32.13,10.88 U2.8 | 43.51,11.43 U$7.P$06 U$7.P$05 | 43.51,11.43 42.81,11.43 C2.1 C8.1 41.51,12 v41.01,12.5 | U$7.P$02 43.53,14.03 43.51,14 43.51,11.43
  Top 0.5: ADC0.16 ADC0.15
  Bottom 0.25: v10.01,35.5 10.01,25 9.01,24 8.01,24 3.01,19 3.01,16 4.01,15 4.01,13.5 5.6,11.91 R8.2 5.63,10.5 9.76,6.38 12.76,6.38 15.13,8.75 15.13,9.75 16.38,11 | v18.01,13.5 16.38,11.88 16.38,11 | v18.01,13.5 R5.2 | v31.63,10.38 31.13,9.88 17.51,9.88 16.88,10.5 16.88,11 | 16.88,11 16.88,11.5 17.51,12.12 18.63,12.12 18.88,11.88 19.26,11.88 22.38,15 22.38,17.88 22.13,18.12 MEMPWR.1 | 16.38,11 16.88,11 | R2.2 33.76,8.25 v31.63,10.38 | R1.2 17.91,13.6 v18.01,13.5 | C20.1 40.01,11 39.01,11 | 39.01,11 C15.1 | 39.01,11 32.26,11 v31.63,10.38 | v31.63,10.38 31.38,10.38 29.76,12 28.26,12 28.01,12.25 28.01,14 28.51,14.5 29.51,14.5 30.01,14 32.51,14 33.01,13.5 40.01,13.5 v41.01,12.5
VDD_CORE  (via drill 0.5, 0.6)
  Top 0.25: v39.01,27.75 36.11,24.85 U$1.VDD_CORE | v34.01,18.62 33.76,18.88 33.76,20.5 32.91,20.5 C12.2 31.58,20.72 C13.2 31.27,21 28.01,21 27.71,21.3 27.71,21.95
  Bottom 0.25: v39.01,27.75 39.01,18.5 38.76,18.25 34.76,18.25 34.38,18.62 v34.01,18.62
(copper drawn outside any net)
  shapes: Top area x1

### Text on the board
Top: V2
Bottom: T Morrison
